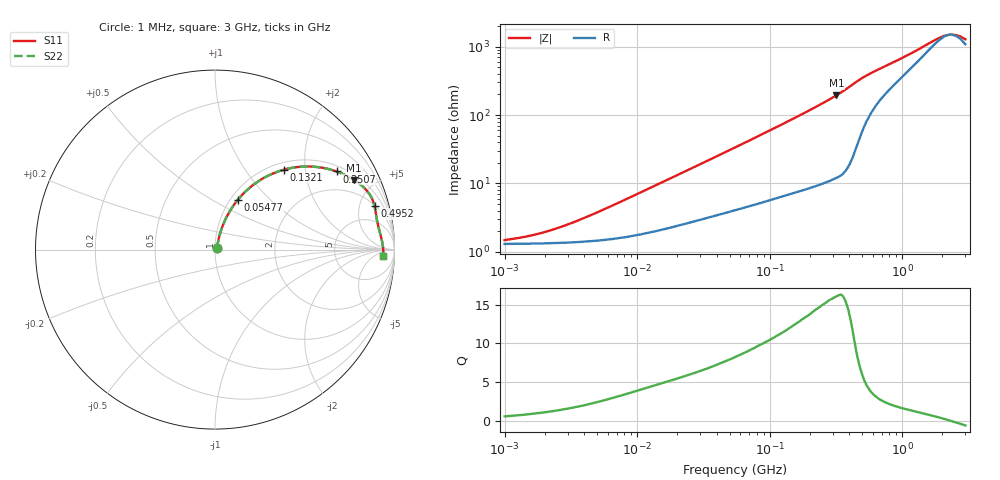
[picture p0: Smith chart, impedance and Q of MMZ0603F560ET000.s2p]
! S-Parameter Data Generated by TDK Corporation
! Copyright(C) 2025 TDK Corporation.
! All Rights Reserved.
! TDK P/N: MMZ0603F560ET000 (Chip Bead)
! Property: |Z|=56ohm at 100MHz
! Size(LxWxT): 0.6x0.3x0.3mm
! Model Type: s2p (Touchstone File Format Version 1.0)
! Frequency: DC=Yes Start=1MHz Stop=3000MHz 202points Log-sweep
! Model Generated on Feb. 6, 2025
! Terms and conditions regarding TDK Simulation Models:
! 1)This simulation model is being provided solely for informational
!  purposes. Please refer to the specifications of the products in
!  terms of detailed characteristics of such products.
! 2)In no event shall TDK Corporation of any of its subsidiaries be
!  liable for any loss or damage arising, directly or indirectly,
!  from any information contained in this simulation model, including,
!  but not limited to loss or damages arising from any inaccuracies,
!  omissions or errors in connection with such information.
! 3)Any and all copyrights on this simulation model are owned by
!  TDK Corporation.  Duplication or redistribution of this simulation
!  model without prior written permission from TDK Corporation
!  is prohibited.
! 4)This simulation model is subject to any modification or change
!  without any prior notice.
! 5)Neither TDK Corporation nor any of its subsidiaries shall make any
!  warranty, express or implied, including but not limited to the
!  correctness, implied warranties of merchantability and fitness for
!  a particular purpose with respect to this simulation models.
! 6)The use of this simulation model shall be deemed to have consented
!  to the terms and conditions hereof.
! Port Assignments:
!  1 ---@@@--- 2
! Applicable Conditions:
!  Temperature = 25 degC
!  DC Bias Current = 0 A
!  Small Signal Operation
# Hz S MA R 50
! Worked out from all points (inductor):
!   201 points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, 1 MHz to 3 GHz, reference 50 ohm
!   read as one part in series: L = 108 nH near 6.831 MHz
!   highest Q = 16.1 at 318.8 MHz (marker M1), where L = 96.6 nH
!   self-resonance near 2.296 GHz
!   S11 on the Smith chart (normalised r, x): 1 MHz: 1.03, +0.01; 54.77 MHz: 1.08, +0.66; 132.1 MHz: 1.13, +1.55; 250.7 MHz: 1.20, +2.96; 495.2 MHz: 2.11, +6.80; 3 GHz: 23, -14
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1000000  0.0146 28.1  0.9871 -0.4  0.9871 -0.4  0.0146 28.1
1377479  0.01607 36.2  0.9871 -0.6  0.9871 -0.6  0.01607 36.2
1897447  0.01856 44.6  0.9869 -0.8  0.9869 -0.8  0.01856 44.6
2613693  0.02244 52.8  0.9866 -1.0  0.9866 -1.0  0.02244 52.8
3900413  0.03017 61.3  0.9858 -1.5  0.9858 -1.5  0.03017 61.3
1.461624e7  0.09626 72.6  0.9756 -5.4  0.9756 -5.4  0.09626 72.6
3.127247e7  0.1894 70.5  0.9537 -10.8  0.9537 -10.8  0.1894 70.5
5.477226e7  0.3065 65.4  0.9156 -17.7  0.9156 -17.7  0.3065 65.4
8.507507e7  0.4353 58.5  0.8572 -25.7  0.8572 -25.7  0.4353 58.5
1.321429e8  0.5894 49.1  0.759 -36.0  0.759 -36.0  0.5894 49.1
1.680187e8  0.6757 43.2  0.6866 -42.4  0.6866 -42.4  0.6757 43.2
2.136344e8  0.7566 37.0  0.6026 -49.0  0.6026 -49.0  0.7566 37.0
2.507343e8  0.805 32.7  0.5422 -53.4  0.5422 -53.4  0.805 32.7
3.188066e8  0.8671 26.5  0.4472 -59.9  0.4472 -59.9  0.8671 26.5
4.0536e8  0.9126 20.2  0.3462 -65.5  0.3462 -65.5  0.9126 20.2
4.951867e8  0.9215 15.3  0.2676 -65.4  0.2676 -65.4  0.9215 15.3
6.296259e8  0.9176 11.4  0.2068 -61.0  0.2068 -61.0  0.9176 11.4
8.005644e8  0.9182 8.6  0.166 -56.3  0.166 -56.3  0.9182 8.6
2.092429e9  0.9365 0.7  0.06465 -10.7  0.06465 -10.7  0.9365 0.7
2.359433e9  0.9379 -0.2  0.06218 3.2  0.06218 3.2  0.9379 -0.2
2.556106e9  0.9381 -0.9  0.06365 12.9  0.06365 12.9  0.9381 -0.9
3e9  0.9376 -2.2  0.073 30.1  0.073 30.1  0.9376 -2.2
